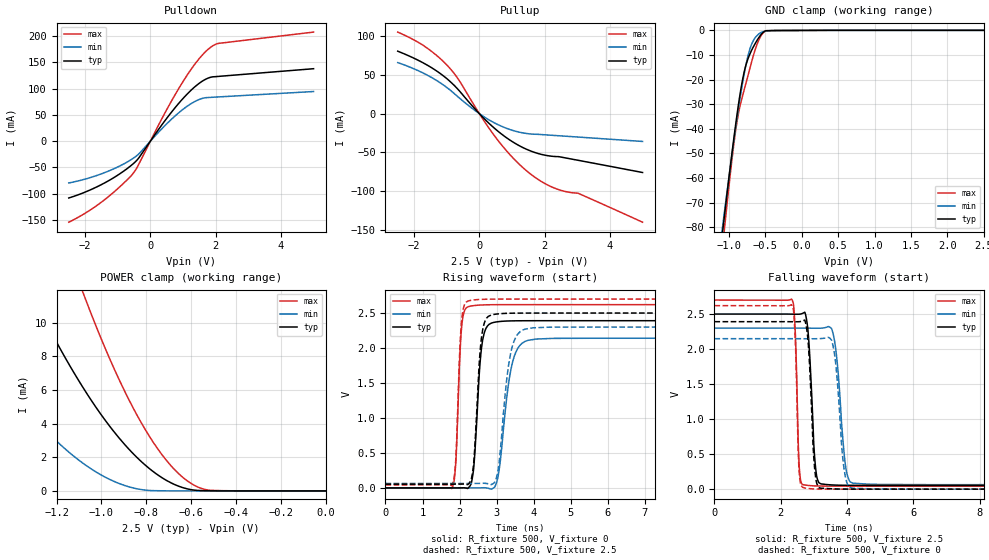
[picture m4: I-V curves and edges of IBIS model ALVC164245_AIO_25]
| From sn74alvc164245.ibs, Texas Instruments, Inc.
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[Model]   ALVC164245_AIO_25
Model_type  I/O
Vinl=0.7
Vinh=1.7
Enable   Active-Low
Vref =   0
Rref =   500
Cref =   30p
Vmeas =   1.25
| variable   typ   min   max
C_comp   8.5pF   NA   NA
| C_pullup   3.31pF   2.77pF   3.78pF
| C_pulldown   3.58pF   2.72pF   4.65pF
| C_tri-state   3.05pF   2.59pF   3.62pF
[Temperature Range]   40   100   -40
| Ambient temperature   25   85   -40
[Voltage range]   2.5   2.3   2.7
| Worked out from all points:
|   slope of the pulldown table from 0 to 0.375 V, typ, clamps not added: 11.4 ohm
|   slope of the pullup table from 0 to 0.375 V, typ, clamps not added: 24.1 ohm
|   GND clamp passes 1 mA (typ) near -0.54 V on its own axis
|   POWER clamp passes 1 mA (typ) near -0.75 V on its own axis
|   rising waveform, R_fixture 500, V_fixture 0: 20-80 % time 165ps typ, 285ps min, 114ps max; typ from 0 V to 2.39 V
|   falling waveform, R_fixture 500, V_fixture 2.5: 20-80 % time 149ps typ, 218ps min, 89.6ps max; typ from 2.5 V to 0.054 V
|   rising waveform, R_fixture 500, V_fixture 2.5: 20-80 % time 158ps typ, 258ps min, 112ps max; typ from 0.054 V to 2.5 V
|   falling waveform, R_fixture 500, V_fixture 0: 20-80 % time 140ps typ, 201ps min, 87.4ps max; typ from 2.39 V to 0 V
[GND Clamp]
| ALVC164245_AIO_25
|   Voltage   I(typ)   I(min)   I(max)
-2.5V     -485mA     -444.7mA   -547.1mA
-1.085V   -81.07mA   -78.95mA   -87.25mA
-1.07V    -77.22mA   -75.45mA   -82.89mA
-1.05V    -72.13mA   -70.82mA   -77.14mA
-915mV    -39.69mA   -41mA      -42.06mA
-870mV    -30.15mA   -31.86mA   -33.77mA
-810mV    -19.51mA   -20.77mA   -26.19mA
-745mV    -12.02mA   -11.07mA   -19.05mA
-695mV    -8.455mA   -6.064mA   -13.44mA
-555mV    -1.559mA   -802.7uA   -1.963mA
-420mV    -88.65uA   -111.7uA   -126.8uA
2.5V      5.797uA    4.08uA     7.268uA
[POWER Clamp]
| ALVC164245_AIO_25
|   Voltage   I(typ)   I(min)   I(max)
-2.5V     55.96mA    34.48mA    87.61mA
-1.675V   23.01mA    11.36mA    38.09mA
-1.49V    16.94mA    7.56mA     28.95mA
-1.3V     11.41mA    4.341mA    20.35mA
-1.085V   6.203mA    1.672mA    11.88mA
-1.07V    5.887mA    1.528mA    11.36mA
-950mV    3.617mA    602.3uA    7.453mA
-825mV    1.777mA    86.65uA    4.109mA
-730mV    784.2uA    8.354uA    2.15mA
-630mV    166.6uA    1.03uA     725uA
-515mV    7.088uA    109.4nA    36.08uA
-31.15fV  1.59nA     14.38nA    4.435nA
[Pulldown]
| ALVC164245_AIO_25
|   Voltage   I(typ)   I(min)   I(max)
-2.5V     -108.1mA   -79.52mA   -154.2mA
-1.98V    -96.42mA   -71.85mA   -136.4mA
-1.5V     -82.63mA   -62.17mA   -116.1mA
-990mV    -64.29mA   -48.83mA   -89.81mA
-540mV    -43.7mA    -33.14mA   -62.24mA
-360mV    -32.29mA   -24.55mA   -44.45mA
385mV     33.85mA    25.78mA    46.64mA
930mV     76.35mA    57.16mA    106.4mA
1.425V    106.7mA    77.45mA    151.6mA
1.825V    121.2mA    83.24mA    177.7mA
2.105V    123.4mA    84.25mA    186.2mA
5V        137.9mA    94.47mA    207.6mA
[Pullup]
| ALVC164245_AIO_25
|   Voltage   I(typ)   I(min)   I(max)
-2.5V     80.42mA    65.73mA    105mA
-1.745V   65.92mA    52.76mA    88.64mA
-975mV    44.3mA     32.98mA    61.73mA
-625mV    29.91mA    20.61mA    43.16mA
-80mV     3.641mA    2.409mA    5.378mA
380mV     -15.75mA   -10.04mA   -23.72mA
975mV     -35.12mA   -21mA      -54.58mA
1.57V     -48.07mA   -26.18mA   -77.81mA
2.245V    -54.97mA   -27.94mA   -94.9mA
2.63V     -56.97mA   -29.04mA   -100.3mA
3.02V     -60.05mA   -30.15mA   -102.4mA
5V        -75.83mA   -35.83mA   -139.8mA
[Ramp]
| ALVC164245_AIO_25
| variable   typ   min   max
dV/dt_r   1.44/1.72E-10   1.29/2.93E-10   1.58/1.18E-10
dV/dt_f   1.48/1.62E-10   1.35/2.30E-10   1.60/9.15E-11
R_load = 500
[Rising Waveform]
| ALVC164245_AIO_25
R_fixture =   500
C_fixture =   0
L_fixture =   0
V_fixture =   0
V_fixture_min = 0
V_fixture_max = 0
|   Time   V(typ)   V(min)   V(max)
0s        176.6pV    3.47nV     104.6nV
1.8ns     -54.46uV   9.349uV    595.2uV
1.9ns     -66.71uV   -6.405uV   377.6mV
2.075ns   1.098mV    -25.38uV   2.392V
2.435ns   696.8mV    -20.02uV   2.609V
2.715ns   2.283V     669.9uV    2.618V
3.03ns    2.376V     137.9mV    2.62V
3.48ns    2.389V     1.887V     2.62V
4.06ns    2.39V      2.128V     2.62V
50ns      2.391V     2.14V      2.62V
[Falling Waveform]
| ALVC164245_AIO_25
R_fixture =   500
C_fixture =   0
L_fixture =   0
V_fixture =   2.5
V_fixture_min = 2.3
V_fixture_max = 2.7
|   Time   V(typ)   V(min)   V(max)
0s        2.5V       2.3V       2.7V
2.345ns   2.499V     2.3V       2.699V
2.44ns    2.498V     2.3V       2.212V
2.57ns    2.499V     2.3V       234.5mV
2.815ns   2.292V     2.299V     54.03mV
3.06ns    263mV      2.297V     45.91mV
3.385ns   66.25mV    2.313V     43.67mV
3.62ns    58.66mV    2.121V     43.16mV
4.195ns   54.74mV    82.12mV    42.81mV
50ns      53.86mV    64.26mV    42.65mV
[Rising Waveform]
| ALVC164245_AIO_25
R_fixture =   500
C_fixture =   0
L_fixture =   0
V_fixture =   2.5
V_fixture_min = 2.3
V_fixture_max = 2.7
|   Time   V(typ)   V(min)   V(max)
0s        53.86mV    64.25mV    42.64mV
1.8ns     53.81mV    64.25mV    43.36mV
1.9ns     53.8mV     64.24mV    428.4mV
2.07ns    54.8mV     64.22mV    2.466V
2.405ns   528mV      64.17mV    2.689V
2.69ns    2.389V     65.88mV    2.697V
3.025ns   2.487V     206.2mV    2.699V
3.44ns    2.498V     2.052V     2.7V
3.985ns   2.5V       2.289V     2.7V
50ns      2.5V       2.3V       2.7V
[Falling Waveform]
| ALVC164245_AIO_25
R_fixture =   500
C_fixture =   0
L_fixture =   0
V_fixture =   0
V_fixture_min = 0
V_fixture_max = 0
|   Time   V(typ)   V(min)   V(max)
0s        2.391V     2.148V     2.62V
2.34ns    2.39V      2.148V     2.622V
2.565ns   2.391V     2.148V     184.3mV
2.805ns   2.201V     2.147V     10.42mV
3.015ns   327.8mV    2.147V     3.432mV
3.215ns   13.57mV    2.15V      1.534mV
3.575ns   4.509mV    2.049V     489.8uV
3.91ns    1.372mV    284.9mV    225.2uV
4.185ns   666.8uV    13.41mV    147.6uV
50ns      6.329uV    9.657uV    7.934uV
